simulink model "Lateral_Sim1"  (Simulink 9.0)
settings: Solver=ode45  StartTime=0.0  StopTime=60  RelTol=1e-3  EnableMultiTasking=on
InitFcn:
  | init_lat;
StopFcn:
  | pl
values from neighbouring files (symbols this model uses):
  d2r = pi/180    (= 0.0174532925199)    [frequ.m]    (also in init_lat.m; pl.m; init.m; freq.m)
undefined symbols (not defined in the file or in its folder): Al, Bl, Cl, Dl, Kpr

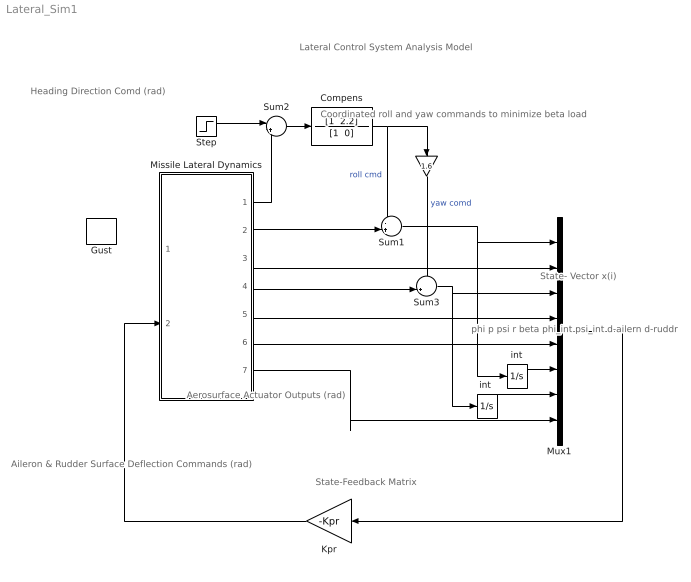
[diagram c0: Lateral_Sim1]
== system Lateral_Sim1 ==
  note: phi p psi r beta phi_int psi_int d-ailern d-ruddr
  note: Heading Direction Comd (rad)
  note: State- Vector x(i)
  note: Aileron & Rudder Surface Deflection Commands (rad)
  note: Aerosurface Actuator Outputs (rad)
  note: Coordinated roll and yaw commands to minimize beta load
  note: State-Feedback Matrix
  note: Lateral Control System Analysis Model
  " " : Gain  Gain=1.6
  Compens : TransferFcn  Numerator="[1  2.2]"  Denominator="[1  0]"
  Gust : DiscretePulseGenerator  PulseType=Time based  Amplitude=40  Period=100  PulseWidth=5  PhaseDelay=10
  Kpr : Gain  Gain=-Kpr  Multiplication=Matrix(K*u)
  Missile Lateral Dynamics : Subsystem
  Mux1 : Mux  Inputs=[1, 1, 1, 1, 1, 1, 1, 2]
  Step : Step  Time=0  After=10*d2r  SampleTime=0
  Sum1 : Sum  Inputs=-+|
  Sum2 : Sum  Inputs=|+-
  Sum3 : Sum  Inputs=-+|
  int : Integrator
  "int " : Integrator
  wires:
  Missile Lateral Dynamics/3(p) -> Mux1/2
  Missile Lateral Dynamics/5(r) -> Mux1/4
  Missile Lateral Dynamics/6(beta-v) -> Mux1/5
  Kpr/1 -> Missile Lateral Dynamics/2(aero)
  Sum1/1 -> Mux1/1, int/1
  Missile Lateral Dynamics/2(phi) -> Sum1/2
  Sum2/1 -> Compens/1
  int/1 -> Mux1/6
  Missile Lateral Dynamics/1(" Head") -> Sum2/2
  Compens/1 -> Sum1/1, " "/1  "roll cmd"
  Missile Lateral Dynamics/4(psi) -> Sum3/2
  Sum3/1 -> Mux1/3, "int "/1
  "int "/1 -> Mux1/7
  " "/1 -> Sum3/1  "yaw comd"
  Missile Lateral Dynamics/7(aeros) -> Mux1/8
  Mux1/1 -> Kpr/1
  Step/1 -> Sum2/1

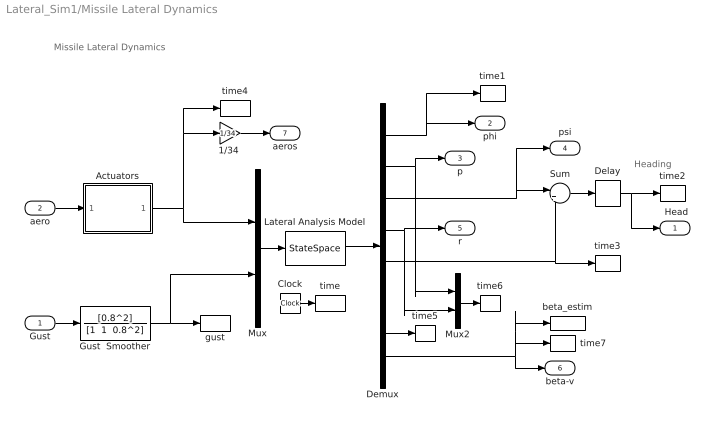
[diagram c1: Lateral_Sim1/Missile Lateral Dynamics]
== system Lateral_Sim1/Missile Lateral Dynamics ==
  note: Heading
  note: Missile Lateral Dynamics
  Gust : Inport
  aero : Inport  Port=2
  "1/34 " : Gain  Gain=1/34
  Actuators : Subsystem
  Clock : Clock
  Delay : TransportDelay  DelayTime=0.5  PadeOrder=2
  Demux : Demux  Outputs=8
  Gust  Smoother : TransferFcn  Numerator=[0.8^2]  Denominator="[1  1  0.8^2]"
  Lateral Analysis Model : StateSpace  A=Al  B=Bl  C=Cl  D=Dl  InitialCondition=0
  Mux : Mux  Inputs=[2, 1]
  Mux2 : Mux  Inputs=2
  Sum : Sum  Inputs=|++
  beta_estim : ToWorkspace  VariableName=betest  SampleTime=-1
  gust : ToWorkspace  VariableName=gust  SampleTime=-1
  time : ToWorkspace  VariableName=time  SampleTime=-1
  time1 : ToWorkspace  VariableName=phi  SampleTime=-1
  time2 : ToWorkspace  VariableName=Head  SampleTime=-1
  time3 : ToWorkspace  VariableName=betai  SampleTime=-1
  time4 : ToWorkspace  VariableName=aeros  SampleTime=-1
  time5 : ToWorkspace  VariableName=Ay  SampleTime=-1
  time6 : ToWorkspace  VariableName=pr  SampleTime=-1
  time7 : ToWorkspace  VariableName=betav  SampleTime=-1
  " Head" : Outport
  phi : Outport  Port=2
  p : Outport  Port=3
  psi : Outport  Port=4
  r : Outport  Port=5
  beta-v : Outport  Port=6
  aeros : Outport  Port=7
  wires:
  Mux/1 -> Lateral Analysis Model/1
  Demux/1 -> time1/1, phi/1
  Demux/2 -> Mux2/1, p/1
  Demux/4 -> Mux2/2, r/1
  Demux/3 -> psi/1, Sum/1
  Demux/5 -> time3/1, Sum/2
  "1/34 "/1 -> aeros/1
  Sum/1 -> Delay/1
  aero/1 -> Actuators/1(deli)
  Clock/1 -> time/1
  Gust/1 -> Gust  Smoother/1
  Demux/7 -> time5/1
  Mux2/1 -> time6/1
  Gust  Smoother/1 -> gust/1, Mux/2
  Lateral Analysis Model/1 -> Demux/1
  Demux/8 -> beta-v/1, beta_estim/1, time7/1
  Delay/1 -> " Head"/1, time2/1
  Actuators/1("delo ") -> Mux/1, time4/1, "1/34 "/1

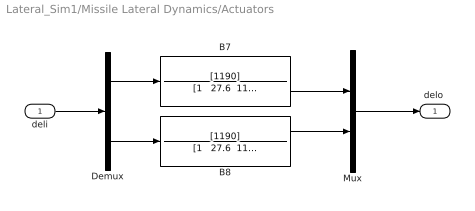
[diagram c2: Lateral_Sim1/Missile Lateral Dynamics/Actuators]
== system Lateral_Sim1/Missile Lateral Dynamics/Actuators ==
  deli : Inport
  B7 : TransferFcn  Numerator=[1190]  Denominator="[1   27.6  1190]"
  B8 : TransferFcn  Numerator=[1190]  Denominator="[1   27.6  1190]"
  Demux : Demux  Outputs=2
  Mux : Mux  Inputs=2
  "delo " : Outport
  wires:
  Mux/1 -> "delo "/1
  B7/1 -> Mux/1
  B8/1 -> Mux/2
  Demux/2 -> B8/1
  Demux/1 -> B7/1
  deli/1 -> Demux/1
